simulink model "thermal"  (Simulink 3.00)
settings: Solver=ode45  SolverMode=SingleTasking  StartTime=0.0  StopTime=1000  RelTol=1e-3  AbsTol=1e-6

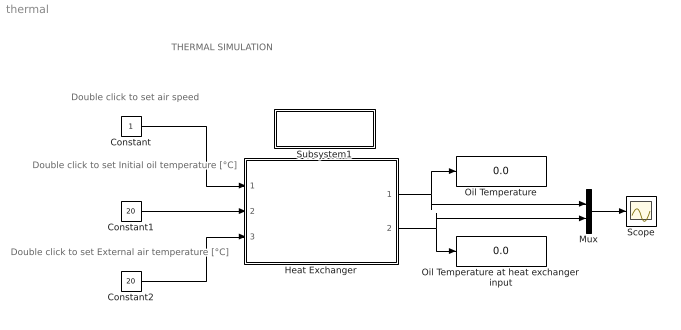
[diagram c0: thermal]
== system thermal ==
  note: Double click to set air speed
  note: Double click to set Initial oil temperature [°C]
  note: Double click to set External air temperature [°C]
  note: THERMAL SIMULATION
  Constant : Constant  Value=1
  Constant1 : Constant  Value=20
  Constant2 : Constant  Value=20
  Heat Exchanger : Subsystem  mask(Heat Exchanger){a_ex=, Row=[ ], Column=[ ], Table=[ ]}
      mask prompts: a_ex "Heat exchange surface [m2]"; Row "Air speed [m/s]  (several values separated by spaces between [ ])"; Column "Oil flow [l/min]  (several values separated by spaces between [ ])"; Table "Exchange coeff. [W/°C m2]  (several values separated by spaces between [ ])"
  Mux : Mux  Inputs=2
  Oil Temperature : Display
  Oil Temperature at heat exchanger input : Display
  Scope : Scope
  Subsystem1 : Subsystem  mask(System data){t_stop=1000, file_name=.thr, h_serb=, a_serb=, oil_mass=, steel_mass=, titan_mass=, all_mass=, oth_mass=}
      mask prompts: t_stop "Simulation stop time [s]"; file_name "Thermal Data file name (simulation name with extention '.thr')"; h_serb "Reservoir exchange coefficient [W/(°C m2)]"; a_serb "Reservoir exchange surface [m2]"; oil_mass "System oil mass [kg]"; steel_mass "System steel mass [kg]"; titan_mass "System titanium mass [kg]"; all_mass "System aluminum mass [kg]"; oth_mass "System other material mass [kg]"
      mask init:
      | fid=fopen(file_name,'r');
      | a=fscanf(fid,'%e %e %e');
      | p_tot=a(1);
      | qm=a(2)/6e4;
      | rho=a(3);
      | status=fclose(fid);
      | ts=num2str(t_stop);
      | set_param(gcs,'StopTime',ts)
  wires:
  Constant2/1 -> Heat Exchanger/3(External air  Temp.)
  Constant1/1 -> Heat Exchanger/2("Initial Oil  Temp. ")
  Constant/1 -> Heat Exchanger/1(v_air)
  Mux/1 -> Scope/1
  Heat Exchanger/1("Oil Temp. ") -> Oil Temperature/1, Mux/1
  Heat Exchanger/2(Oil Temp. at h. e. input) -> Oil Temperature at heat exchanger input/1, Mux/2

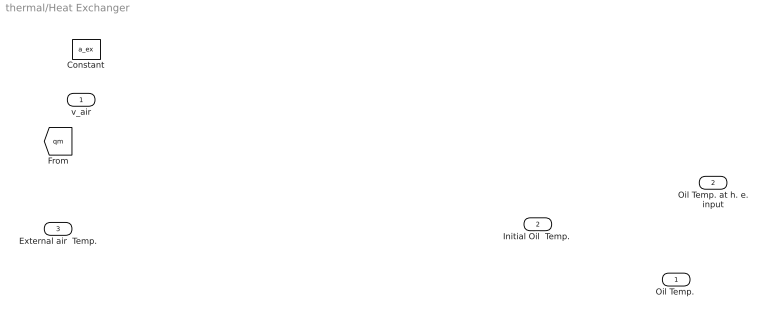
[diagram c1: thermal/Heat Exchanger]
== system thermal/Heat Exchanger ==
  v_air : Inport  Port=1  PortWidth=-1  SampleTime=-1  DataType=auto
  "Initial Oil  Temp. " : Inport  Port=2  PortWidth=-1  SampleTime=-1  DataType=auto
  External air  Temp. : Inport  Port=3  PortWidth=-1  SampleTime=-1  DataType=auto
  Constant : Constant  Value=a_ex
  "Oil Temp. " : Outport  Port=1
  Oil Temp. at h. e. input : Outport  Port=2
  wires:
  ? -> Oil Temp. at h. e. input/1

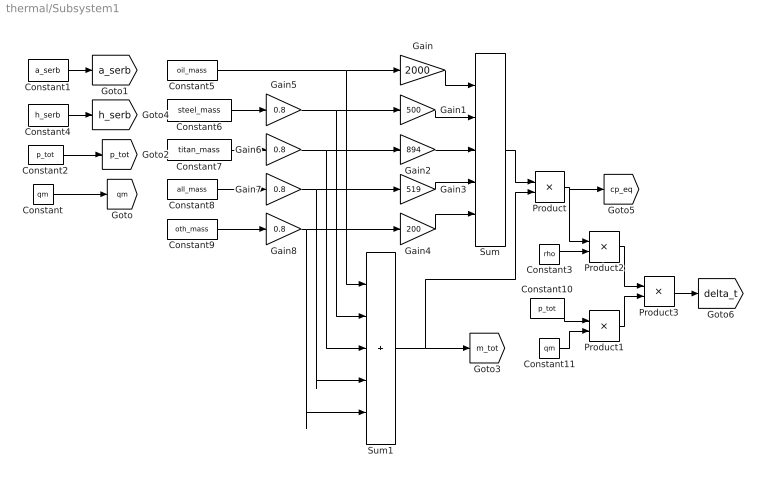
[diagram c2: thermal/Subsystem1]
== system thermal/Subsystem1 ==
  Constant : Constant  Value=qm
  Constant1 : Constant  Value=a_serb
  Constant10 : Constant  Value=p_tot
  Constant11 : Constant  Value=qm
  Constant2 : Constant  Value=p_tot
  Constant3 : Constant  Value=rho
  Constant4 : Constant  Value=h_serb
  Constant5 : Constant  Value=oil_mass
  Constant6 : Constant  Value=steel_mass
  Constant7 : Constant  Value=titan_mass
  Constant8 : Constant  Value=all_mass
  Constant9 : Constant  Value=oth_mass
  Gain : Gain  Gain=2000  SaturateOnIntegerOverflow=on
  Gain1 : Gain  Gain=500  SaturateOnIntegerOverflow=on
  Gain2 : Gain  Gain=894  SaturateOnIntegerOverflow=on
  Gain3 : Gain  Gain=519  SaturateOnIntegerOverflow=on
  Gain4 : Gain  Gain=200  SaturateOnIntegerOverflow=on
  Gain{5..8} (4 alike) : Gain  Gain=0.8  SaturateOnIntegerOverflow=on
  Product : Product  Inputs=*/  SaturateOnIntegerOverflow=on
  Product1 : Product  Inputs=*/  SaturateOnIntegerOverflow=on
  Product2 : Product  Inputs=2  SaturateOnIntegerOverflow=on
  Product3 : Product  Inputs=/*  SaturateOnIntegerOverflow=on
  Sum : Sum  Inputs=+++++  SaturateOnIntegerOverflow=on
  Sum1 : Sum  Inputs=+++++  SaturateOnIntegerOverflow=on
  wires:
  Constant1/1 -> [a_serb]
  Constant6/1 -> Gain5/1
  Constant7/1 -> Gain6/1
  Constant9/1 -> Gain8/1
  Constant8/1 -> Gain7/1
  Constant5/1 -> Gain/1, Sum1/1
  Gain5/1 -> Gain1/1, Sum1/2
  Gain6/1 -> Gain2/1, Sum1/3
  Gain7/1 -> Gain3/1, Sum1/4
  Gain8/1 -> Gain4/1, Sum1/5
  Product1/1 -> Product3/2
  Gain/1 -> Sum/1
  Gain1/1 -> Sum/2
  Gain2/1 -> Sum/3
  Gain3/1 -> Sum/4
  Gain4/1 -> Sum/5
  Sum/1 -> Product/1
  Product/1 -> Product2/1, [cp_eq]
  Product2/1 -> Product3/1
  Constant2/1 -> [p_tot]
  Constant4/1 -> [h_serb]
  Constant/1 -> [qm]
  Product3/1 -> [delta_t]
  Sum1/1 -> [m_tot], Product/2
  Constant3/1 -> Product2/2
  Constant10/1 -> Product1/1
  Constant11/1 -> Product1/2
